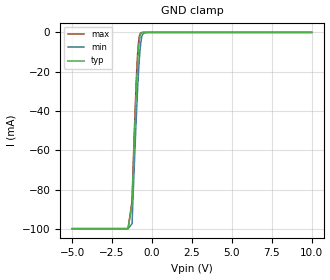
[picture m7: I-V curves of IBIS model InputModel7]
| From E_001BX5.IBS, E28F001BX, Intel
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|*********************Input Model 7*******************************
[Model]   InputModel7
Model_type   Input
|   Model for RP# pin
Vinl = 0.8V
Vinh = 2.0V
|Variable   Typ   Min   Max
C_comp   9.13p   7.20p   11.06p
[Voltage Range]   5.0V   4.5V   5.5V
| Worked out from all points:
|   GND clamp passes 1 mA (typ) near -0.71 V on its own axis
[GND_clamp]
|Voltage   I(typ)   I(min)   I(max)
-5V       -99.85mA   -99.85mA   -99.85mA
-1.5V     -99.85mA   -99.85mA   -99.85mA
-1.25V    -87.38mA   -97.43mA   -85.99mA
-1.1V     -52.92mA   -66.15mA   -49.26mA
-950mV    -22.84mA   -37.27mA   -18.3mA
-900mV    -14.89mA   -28.72mA   -10.7mA
-850mV    -8.713mA   -21.12mA   -5.404mA
-800mV    -4.335mA   -14.4mA    -2.205mA
-700mV    -677.6uA   -5.134mA   -232.3uA
-600mV    -70.5uA    -1.252mA   -25.04uA
-250mV    0A         0A         0A
10V       0A         0A         0A
[Power_clamp]
| Input buffer circuits of this product do not intrinisically
| require a [Power_clamp] defintion.  This zero current
| [Power_clamp] table is provided for compatibility with
| some IBIS parsers.
|Voltage   I(typ)   I(min)   I(max)
-5V       0A         0A         0A
0V        0A         0A         0A
5V        0A         0A         0A
10V       0A         0A         0A
